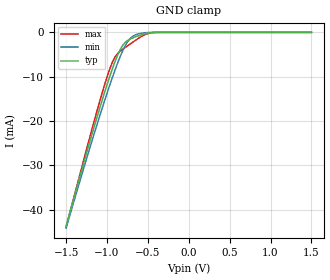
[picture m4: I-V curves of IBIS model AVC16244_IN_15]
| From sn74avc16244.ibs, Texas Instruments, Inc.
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[Model]   AVC16244_IN_15
Model_type  Input
Vinl=0.49
Vinh=1.04
| variable   typ   min   max
C_comp   4.10pF   3.26pF   5.52pF
[Temperature Range]   40   100   -40
| Ambient temperature   25   85   -40
[Voltage range]   1.5   1.4   1.6
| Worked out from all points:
|   GND clamp passes 1 mA (typ) near -0.65 V on its own axis
[GND Clamp]
| AVC16244_IN_15
|   Voltage   I(typ)   I(min)   I(max)
-1.5V     -43.67mA   -44.19mA   -44.05mA
-1.16V    -21.52mA   -23.09mA   -20.25mA
-1.05V    -14.77mA   -16.61mA   -13.1mA
-970mV    -10.15mA   -12.11mA   -8.465mA
-900mV    -6.506mA   -8.414mA   -5.523mA
-825mV    -3.453mA   -4.886mA   -4.059mA
-755mV    -1.927mA   -2.335mA   -3.135mA
-695mV    -1.315mA   -1.035mA   -2.359mA
-635mV    -882uA     -451.7uA   -1.573mA
-550mV    -386.4uA   -123.6uA   -652.1uA
-430mV    -20.24uA   -13.73uA   -29.52uA
1.5V      199.2pA    687.4pA    10.54pA
